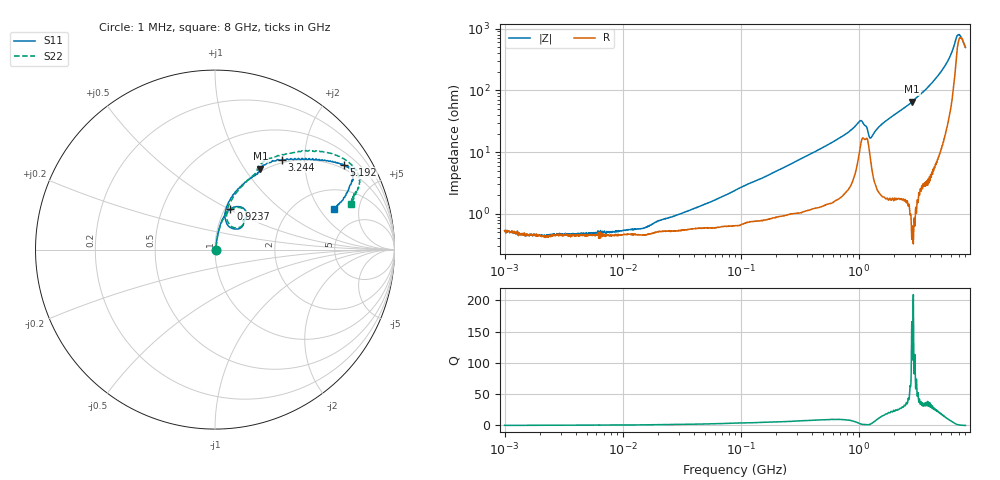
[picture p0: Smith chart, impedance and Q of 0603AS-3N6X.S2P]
!s-Parameter Generated by FASTRON Sdn. Bhd.
!FASTRON P/N : 0603AS-3N6X
!Keysight Technologies: E5071C_MY46733604_B.14.02
!Date: Tue Oct 24 10:24:57 2023
!Version  :Rev01  Tue Oct 24 10:24:57 2023
!Data & Calibration Information:
!Freq  S11:SOLT2(ON)  S21:SOLT2(ON)  S12:SOLT2(ON)  S22:SOLT2(ON)
!PortZ  Port1:50+j0  Port2:50+j0
!When reading reference impedance value at option line is always used.
! Remarks : This data is being provided solely for informational purposes.
# Hz S dB R 50
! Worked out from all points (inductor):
!   1601 points, 1 MHz to 8 GHz, reference 50 ohm
!   read as one part in series: L = 4.1 nH near 73.11 MHz
!   highest Q = 73.9 at 2.839 GHz (marker M1), where L = 3.69 nH
!   self-resonance near 7.633 GHz
!   S11 on the Smith chart (normalised r, x): 1 MHz: 1.01, -0.00; 923.7 MHz: 1.06, +0.51; 3.244 GHz: 0.95, +1.56; 5.192 GHz: 0.86, +3.13; 8 GHz: 3.11, +2.77
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1000000  -44.72 -3.2  -0.04 -0.1  -0.04 -0.0  -44.80 1.2
1541011  -48.51 -9.2  -0.04 -0.1  -0.04 -0.0  -45.58 -20.3
2211112  -47.57 9.3  -0.04 -0.0  -0.04 -0.1  -49.94 24.9
2905262  -47.69 11.8  -0.05 -0.1  -0.05 -0.1  -48.15 9.4
4479405  -46.70 16.7  -0.04 -0.1  -0.05 -0.1  -48.19 21.8
8407329  -46.15 26.1  -0.04 -0.1  -0.04 -0.2  -46.45 28.2
1.483728e7  -51.71 30.2  -0.04 -0.3  -0.05 -0.3  -43.35 31.5
1.587214e7  -50.68 36.4  -0.04 -0.3  -0.05 -0.3  -43.15 34.5
2.00676e7  -43.03 47.5  -0.04 -0.4  -0.05 -0.3  -42.02 52.4
8.994653e7  -32.53 74.6  -0.06 -1.4  -0.07 -1.4  -32.83 73.1
4.006501e8  -20.43 79.3  -0.16 -5.3  -0.17 -5.3  -20.43 78.7
9.236575e8  -12.33 69.2  -0.68 -13.5  -0.69 -13.5  -12.35 68.0
1.047189e9  -11.20 51.6  -1.52 -13.9  -1.53 -13.9  -11.36 50.5
1.264475e9  -16.23 63.3  -0.75 -7.9  -0.76 -8.0  -15.86 59.9
1.7949e9  -9.81 71.7  -0.77 -18.6  -0.78 -18.7  -9.82 70.3
2.839031e9  -5.74 60.7  -2.34 -33.3  -2.36 -33.4  -5.69 62.2
3.244011e9  -4.08 53.3  -2.98 -36.0  -2.99 -36.0  -4.06 56.4
4.034495e9  -2.59 42.8  -4.84 -44.9  -4.83 -45.0  -2.50 47.2
5.192391e9  -1.31 33.3  -8.86 -52.6  -8.85 -52.7  -1.20 36.2
5.995147e9  -1.12 30.0  -12.85 -53.3  -12.84 -53.4  -0.92 30.1
6.959019e9  -1.63 25.2  -19.79 -19.1  -19.78 -19.5  -1.30 22.6
8e9  -3.07 18.7  -16.59 25.3  -16.58 24.9  -1.93 18.3
